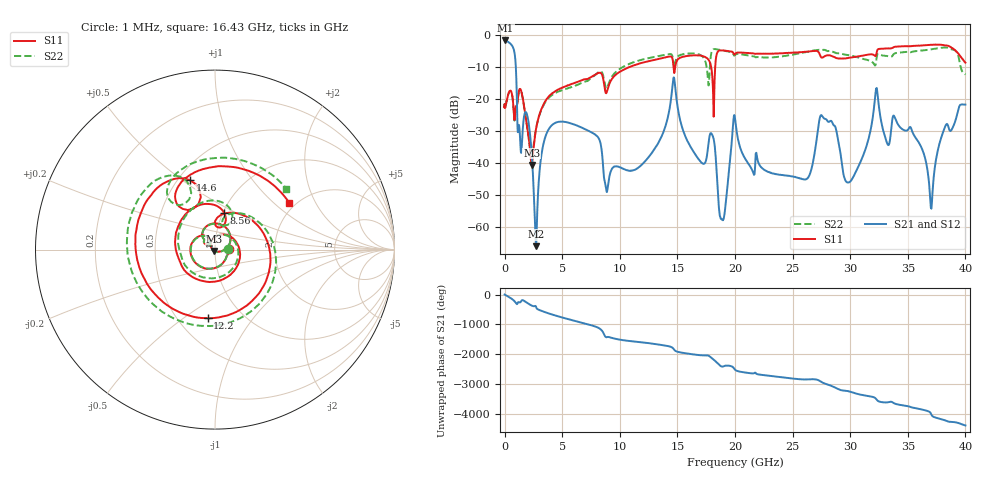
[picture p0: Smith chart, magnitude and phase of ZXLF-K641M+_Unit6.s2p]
! Mini-Circuits
! S2P DATA File Format
! Type: LOW PASS FILTER
! Model: ZXLF-K641M+
! All S Parameters are in dB deg format
! TEST CONDITIONS: INPUT POWER = 0 dBm - Unit-6
# GHZ S RI R 50.0
! FREQ.GHZ  S11RE  S11IM  S21RE  S21IM  S12RE  S12IM  S22RE  S22IM
!; PortSelection: Port_12
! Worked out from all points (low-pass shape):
!   1320 points, 1 MHz to 40 GHz, reference 50 ohm
!   highest |S21| = -1.56 dB at 60 MHz (marker M1); lowest = -65.9 dB at 2.74 GHz (marker M2)
!   |S21| within 3 dB of the highest: start of sweep to 809.6 MHz
!   lowest |S11| = -40.5 dB at 2.36 GHz (marker M3), VSWR 1.02, Z = 49.5 - j0.792 ohm
!   |S11| at or under -10 dB: start of sweep to 10.74 GHz; 14.67 GHz to 14.8 GHz (138.5 MHz wide, 0.94 % of centre); 17.94 GHz to 18.28 GHz (340.9 MHz wide, 1.88 % of centre)
!   |S22| runs from -39.1 to -3.7 dB; largest |S21 - S12| = 0.0022
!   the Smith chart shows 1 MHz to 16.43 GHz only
!   S11 on the Smith chart (normalised r, x): 1 MHz: 1.16, +0.01; 8.56 GHz: 1.02, +0.43; 12.2 GHz: 0.69, -0.62; 14.6 GHz: 0.58, +0.53; 16.43 GHz: 1.85, +1.26
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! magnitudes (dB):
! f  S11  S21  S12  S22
! 1 MHz  -22.4  -1.6  -1.6  -22.5
! 60 MHz  -22.6  -1.6  -1.6  -22.5
! 840 MHz  -26.2  -5.0  -5.0  -26.3
! 1.4 GHz  -16.9  -35.9  -36.0  -17.1
! 2.36 GHz  -40.5  -37.4  -37.4  -38.9
! 2.74 GHz  -29.1  -65.9  -65.7  -28.9
! 3.7 GHz  -19.7  -30.2  -30.2  -20.0
! 6.68 GHz  -14.0  -28.8  -28.8  -14.9
! 8.56 GHz  -13.6  -41.5  -41.4  -12.6
! 12.2 GHz  -8.3  -39.3  -39.4  -7.3
! 13.35 GHz  -7.4  -33.5  -33.6  -6.5
! 14.6 GHz  -7.7  -14.8  -14.8  -6.9
! 16.43 GHz  -6.2  -36.5  -36.5  -5.6
! 18.02 GHz  -12.7  -31.1  -31.2  -4.6
! 18.9 GHz  -4.7  -57.6  -57.6  -4.7
! 20.05 GHz  -5.6  -27.4  -27.4  -6.0
! 26.7 GHz  -4.9  -40.8  -40.9  -4.8
! 27.6 GHz  -6.9  -25.3  -25.4  -4.5
! 29.8 GHz  -7.0  -46.0  -46.1  -6.1
! 33.35 GHz  -4.0  -34.2  -34.3  -6.5
! 37.05 GHz  -2.9  -54.2  -54.2  -4.3
! 40 GHz  -8.5  -21.6  -21.6  -12.2
